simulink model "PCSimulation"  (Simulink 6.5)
settings: Solver=FixedStepDiscrete  SolverMode=SingleTasking  StartTime=0.0  StopTime=inf  FixedStep=samplePeriod  RelTol=1e-3  AbsTol=1e-6
PreLoadFcn:
  | initialize
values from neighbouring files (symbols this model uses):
  accelCanon = 9810    [initialize.m]
  accelFreq = inf    [initialize.m]
  actParams = [	bulkModulus   * pressCanon    [initialize.m]    (also in Copy of initialize.m)
  aFnd = [1]    [initialize.m]
  aFwd = [1]    [initialize.m]
  aLpf = [1]    [randth.m]
  bFnd = [1]    [initialize.m]
  bFwd = [1]    [initialize.m]
  bLpf = [1]    [randth.m]
  displFreq = inf    [initialize.m]
  flowCanon = 1.666667e+04    (= 16666.67)    [initialize.m]    (also in Copy of initialize.m)
  forceCanon = 1    [initialize.m]    (also in Copy of initialize.m)
  forceFreq = inf    [initialize.m]
  friction = 5			 				* 0.155000	 				* 0.00444822 				* area1    (= 2.71252900422)    [initialize.m]
  fsamp = 1 / samplePeriod    (= 1024)    [initialize.m]    (also in rampth.m = 1 / deltaT; randth.m = 1 / deltaT; rspect.m = 1.0 / tsamp; Copy of initialize.m)
  gasConstant = 1.8    [initialize.m]    (also in Copy of initialize.m)
  invFoundMass = 0.0    (= 0)    [initialize.m]
  invRigidMass = 0.0    (= 0)    [initialize.m]
  lengthCanon = 1    [initialize.m]    (also in Copy of initialize.m)
  maxDispl = ( (stroke2 + endLength2) * lengthCanon)'    [initialize.m]    (also in Copy of initialize.m)
  maxOilVolume = volume * (1 - (precharge/supplyPress)^(1/gasConstant))    (= 211.391477114)    [initialize.m]    (also in Copy of initialize.m)
  maxVeloc = ( (maxFlow' * flowCanon ./ (area1 * areaCanon)) / velocCanon)'    [initialize.m]    (also in rampth.m = 2 * maxDispl / (nVeloc * deltaT); Copy of initialize.m)
  minDispl = (-(stroke1 + endLength1) * lengthCanon)'    [initialize.m]    (also in Copy of initialize.m)
  minVeloc = (-(maxFlow' * flowCanon ./ (area2 * areaCanon)) / velocCanon)'    [initialize.m]    (also in Copy of initialize.m)
  nAdcU = 6    [initialize.m]    (also in Copy of initialize.m)
  nUDPInp = 1+6*nAct+nAdcU+nDucU+nEncU+nDout    (= 46)    [initialize.m]    (also in Copy of initialize.m)
  nUDPOut = 1+7*nAct+nAdcU+nDucU+nEncU+nDinp    (= 51)    [initialize.m]    (also in Copy of initialize.m)
  precharge = 3000		 				* 6.894757e-03    (= 20.684271)    [initialize.m]    (also in Copy of initialize.m)
  pumpFlow = 1e20    (= 1e+20)    [initialize.m]    (also in Copy of initialize.m)
  returnPress = 3			 				* 0.1    (= 0.3)    [initialize.m]    (also in Copy of initialize.m)
  samplePeriod = controlPeriod/upsampleFactor    (= 0.0009765625)    [initialize.m]    (also in viewer.m = eval(getHeaderValue(header, 'DELTA_T')); Copy of initialize.m)
  supplyPress = 280		 				* 0.1    (= 28)    [initialize.m]    (also in Copy of initialize.m)
  upsampleFactor = 1    [initialize.m]    (also in Copy of initialize.m)
  velocCanon = 1    [initialize.m]    (also in Copy of initialize.m)
  volume = 15.15		 				+ (  45		 				    * 2		 				   + 30		 				    * 6 )	 				* 5    (= 1365.15)    [initialize.m]    (also in quake.m = volume / 231.0; Copy of initialize.m)
  volumeCanon = 1e+06    (= 1000000)    [initialize.m]    (also in Copy of initialize.m)
  yieldDispl = 1.0    (= 1)    [initialize.m]
undefined symbols (not defined in the file or in its folder): DiscIntNeverNeededParam
libraries: simulink x1

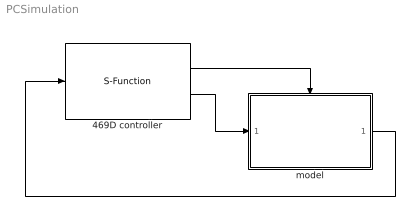
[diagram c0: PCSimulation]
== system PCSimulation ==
  469D controller : S-Function  FunctionName=ConnectUdpSimulink  Parameters=5002,nUDPInp,nUDPOut,upsampleFactor
  model : Subsystem  TreatAsAtomicUnit=on
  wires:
  model/1(out) -> 469D controller/1
  469D controller/1 -> model/Trigger
  469D controller/2 -> model/1(inp)

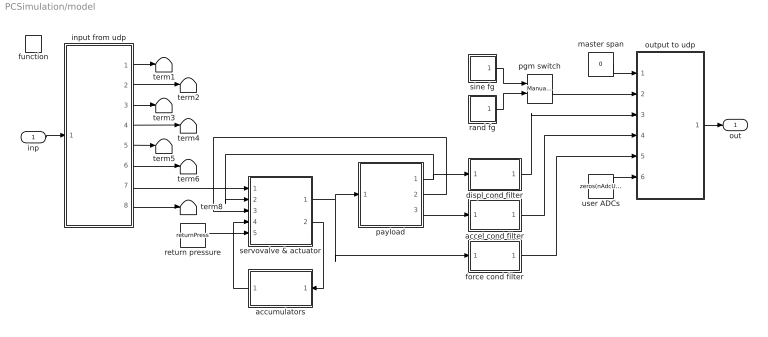
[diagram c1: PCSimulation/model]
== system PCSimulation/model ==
  inp : Inport
  function : TriggerPort  TriggerType=function-call
  accel cond filter : Subsystem  mask{freq3dB=accelFreq, fsamp=fsamp}
      mask prompts: freq3dB "3 dB cutoff frequency (inf, 500, 300, 100, 50 Hz)"; fsamp "Sampling frequency (Hz)"
      mask init:
      | if isempty(freq3dB)
      | 	freq3dB = fsamp;
      | elseif freq3dB == 500
      | 	freq3dB = 485;
      | elseif freq3dB == 300
      | 	freq3dB = 204.9;
      | elseif freq3dB == 100
      | 	freq3dB = 56.5;
      | elseif freq3dB == 50
      | 	freq3dB = 27.8;
      | else
      | 	freq3dB = fsamp;
      | end
      | if freq3dB > fsamp/2
      | 	a = [1];
      | 	b = [1];
      | else
      | 	[b, a] = ellip(4, 0.001, 60.0, 2*freq3dB/fsamp);
      | end
  accumulators : Subsystem  Orientation=left
  displ cond filter : Subsystem  mask{freq3dB=displFreq, fsamp=fsamp}
      mask prompts: freq3dB "3 dB cutoff frequency (inf, 500, 300, 100, 50 Hz)"; fsamp "Sampling frequency (Hz)"
      mask init:
      | if isempty(freq3dB)
      | 	freq3dB = fsamp;
      | elseif freq3dB == 500
      | 	freq3dB = 485;
      | elseif freq3dB == 300
      | 	freq3dB = 204.9;
      | elseif freq3dB == 100
      | 	freq3dB = 56.5;
      | elseif freq3dB == 50
      | 	freq3dB = 27.8;
      | else
      | 	freq3dB = fsamp;
      | end
      | if freq3dB > fsamp/2
      | 	a = [1];
      | 	b = [1];
      | else
      | 	[b, a] = ellip(4, 0.001, 60.0, 2*freq3dB/fsamp);
      | end
  force cond filter : Subsystem  mask{freq3dB=forceFreq, fsamp=fsamp}
      mask prompts: freq3dB "3 dB cutoff frequency (inf, 500, 300, 100, 50 Hz)"; fsamp "Sampling frequency (Hz)"
      mask init:
      | if isempty(freq3dB)
      | 	freq3dB = fsamp;
      | elseif freq3dB == 500
      | 	freq3dB = 485;
      | elseif freq3dB == 300
      | 	freq3dB = 204.9;
      | elseif freq3dB == 100
      | 	freq3dB = 56.5;
      | elseif freq3dB == 50
      | 	freq3dB = 27.8;
      | else
      | 	freq3dB = fsamp;
      | end
      | if freq3dB > fsamp/2
      | 	a = [1];
      | 	b = [1];
      | else
      | 	[b, a] = ellip(4, 0.001, 60.0, 2*freq3dB/fsamp);
      | end
  input from udp : Subsystem
  master span : Constant  Value=0  OutDataType=sfix(16)  ConRadixGroup=Use specified scaling  OutScaling=2^0  SampleTime=inf  FramePeriod=inf
  output to udp : Subsystem
  payload : Subsystem
  pgm switch : simulink/Signal Routing/Manual Switch  SystemSampleTime=-1  sw=0  action=0
  rand fg : Subsystem  mask(Sine Function Generator){ampl=1, bw=10, spanInterval=1, samplePeriod=samplePeriod}
      mask prompts: ampl "RMS amplitude"; bw "Bandwidth (Hz)"; spanInterval "Span interval (sec)"; samplePeriod "Sample period (sec)"
      mask init:
      | gain = ampl*sqrt(3)*sqrt(1/(2*samplePeriod*bw));
  return pressure : Constant  Value=returnPress  OutDataType=sfix(16)  ConRadixGroup=Use specified scaling  OutScaling=2^0  SampleTime=inf  FramePeriod=inf
  servovalve & actuator : Subsystem  mask(Actuator){params=actParams}
      mask prompts: params "Parameter vector"
  sine fg : Subsystem  mask(Sine Function Generator){ampl=1, freq=1, spanInterval=1, samplePeriod=samplePeriod}
      mask prompts: ampl "Amplitude"; freq "Frequency (Hz)"; spanInterval "Span interval (sec)"; samplePeriod "Sample period (sec)"
  term{1..6,8} (7 alike) : Terminator
  user ADCs : Constant  Value=zeros(nAdcU, 1)  OutDataType=sfix(16)  ConRadixGroup=Use specified scaling  OutScaling=2^0  SampleTime=inf  FramePeriod=inf
  out : Outport
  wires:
  servovalve & actuator/2(flow) -> accumulators/1(flow)
  accumulators/1(press) -> servovalve & actuator/4(spl press)
  return pressure/1 -> servovalve & actuator/5(rtn press)
  payload/1(displ) -> displ cond filter/1(inp), servovalve & actuator/2(displ)
  payload/2(veloc) -> servovalve & actuator/3(veloc)
  servovalve & actuator/1(force) -> payload/1(force), force cond filter/1(inp)
  payload/3(accel) -> accel cond filter/1(inp)
  inp/1 -> input from udp/1(inp)
  output to udp/1(out) -> out/1
  user ADCs/1 -> output to udp/6(user adcs)
  input from udp/1(master span) -> term1/1
  input from udp/2(ref) -> term2/1
  input from udp/3(displ fbk) -> term3/1
  input from udp/4(veloc fbk) -> term4/1
  input from udp/5(accel fbk) -> term5/1
  input from udp/6(force fbk) -> term6/1
  input from udp/7(valve cmd) -> servovalve & actuator/1(cmd)
  force cond filter/1(out) -> output to udp/5(force fbk)
  displ cond filter/1(out) -> output to udp/3(displ fbk)
  master span/1 -> output to udp/1(master span)
  sine fg/1(out) -> pgm switch/1
  rand fg/1(out) -> pgm switch/2
  pgm switch/1 -> output to udp/2(ref)
  input from udp/8(user adcs) -> term8/1
  accel cond filter/1(out) -> output to udp/4(accel fbk)

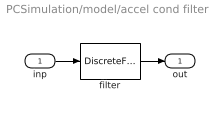
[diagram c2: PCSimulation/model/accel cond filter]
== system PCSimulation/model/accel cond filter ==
  inp : Inport
  filter : DiscreteFilter  Numerator=b  Denominator=a  SampleTime=-1
  out : Outport
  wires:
  inp/1 -> filter/1
  filter/1 -> out/1

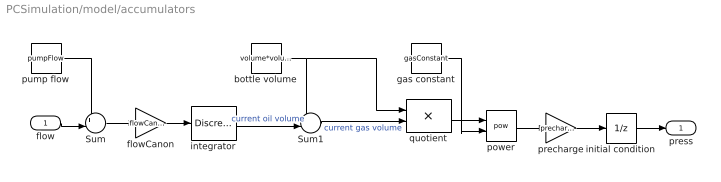
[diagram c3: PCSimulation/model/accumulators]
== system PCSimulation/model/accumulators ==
  flow : Inport
  Sum : Sum  Inputs=+-|
  Sum1 : Sum  Inputs=+-|
  bottle volume : Constant  Value=volume*volumeCanon  OutDataType=sfix(16)  ConRadixGroup=Use specified scaling  OutScaling=2^0  SampleTime=inf  FramePeriod=inf
  flowCanon : Gain  Gain=flowCanon
  gas constant : Constant  Value=gasConstant  OutDataType=sfix(16)  ConRadixGroup=Use specified scaling  OutScaling=2^0  SampleTime=inf  FramePeriod=inf
  initial condition : UnitDelay  X0=supplyPress  SampleTime=-1
  integrator : DiscreteIntegrator  InitialCondition=maxOilVolume*volumeCanon  SampleTime=-1  LimitOutput=on  UpperSaturationLimit=maxOilVolume*volumeCanon  LowerSaturationLimit=0  ICPrevOutput=DiscIntNeverNeededParam  ICPrevScaledInput=DiscIntNeverNeededParam
  power : Math  Operator=pow
  precharge : Gain  Gain=precharge
  pump flow : Constant  Value=pumpFlow  OutDataType=sfix(16)  ConRadixGroup=Use specified scaling  OutScaling=2^0  SampleTime=inf  FramePeriod=inf
  quotient : Product  Inputs=*/
  press : Outport
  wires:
  initial condition/1 -> press/1
  flowCanon/1 -> integrator/1
  flow/1 -> Sum/2
  integrator/1 -> Sum1/2  "current oil volume"
  quotient/1 -> power/1
  Sum1/1 -> quotient/2  "current gas volume"
  precharge/1 -> initial condition/1
  power/1 -> precharge/1
  gas constant/1 -> power/2
  bottle volume/1 -> quotient/1, Sum1/1
  Sum/1 -> flowCanon/1
  pump flow/1 -> Sum/1

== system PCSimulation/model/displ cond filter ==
  inp : Inport
  filter : DiscreteFilter  Numerator=b  Denominator=a  SampleTime=-1
  out : Outport
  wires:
  inp/1 -> filter/1
  filter/1 -> out/1

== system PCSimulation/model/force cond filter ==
  inp : Inport
  filter : DiscreteFilter  Numerator=b  Denominator=a  SampleTime=-1
  out : Outport
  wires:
  filter/1 -> out/1
  inp/1 -> filter/1

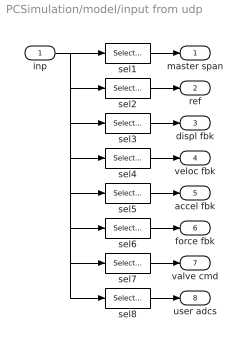
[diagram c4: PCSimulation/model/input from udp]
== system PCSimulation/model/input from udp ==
  inp : Inport
  sel1 : Selector  InputType=Vector  ElementSrc=Internal  Elements=1  RowSrc=Internal  Rows=1  ColumnSrc=Internal  Columns=1  InputPortWidth=nUDPOut  IndexIsStartValue=off
  sel2 : Selector  InputType=Vector  ElementSrc=Internal  Elements=2  RowSrc=Internal  Rows=1  ColumnSrc=Internal  Columns=1  InputPortWidth=nUDPOut  IndexIsStartValue=off
  sel3 : Selector  InputType=Vector  ElementSrc=Internal  Elements=3  RowSrc=Internal  Rows=1  ColumnSrc=Internal  Columns=1  InputPortWidth=nUDPOut  IndexIsStartValue=off
  sel4 : Selector  InputType=Vector  ElementSrc=Internal  Elements=4  RowSrc=Internal  Rows=1  ColumnSrc=Internal  Columns=1  InputPortWidth=nUDPOut  IndexIsStartValue=off
  sel5 : Selector  InputType=Vector  ElementSrc=Internal  Elements=5  RowSrc=Internal  Rows=1  ColumnSrc=Internal  Columns=1  InputPortWidth=nUDPOut  IndexIsStartValue=off
  sel6 : Selector  InputType=Vector  ElementSrc=Internal  Elements=6  RowSrc=Internal  Rows=1  ColumnSrc=Internal  Columns=1  InputPortWidth=nUDPOut  IndexIsStartValue=off
  sel7 : Selector  InputType=Vector  ElementSrc=Internal  Elements=7  RowSrc=Internal  Rows=1  ColumnSrc=Internal  Columns=1  InputPortWidth=nUDPOut  IndexIsStartValue=off
  sel8 : Selector  InputType=Vector  ElementSrc=Internal  Elements=8:12  RowSrc=Internal  Rows=1  ColumnSrc=Internal  Columns=1  InputPortWidth=nUDPOut  IndexIsStartValue=off
  master span : Outport
  ref : Outport  Port=2
  displ fbk : Outport  Port=3
  veloc fbk : Outport  Port=4
  accel fbk : Outport  Port=5
  force fbk : Outport  Port=6
  valve cmd : Outport  Port=7
  user adcs : Outport  Port=8
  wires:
  inp/1 -> sel1/1, sel2/1, sel3/1, sel4/1, sel5/1, sel6/1, sel7/1, sel8/1
  sel7/1 -> valve cmd/1
  sel6/1 -> force fbk/1
  sel5/1 -> accel fbk/1
  sel4/1 -> veloc fbk/1
  sel3/1 -> displ fbk/1
  sel2/1 -> ref/1
  sel1/1 -> master span/1
  sel8/1 -> user adcs/1

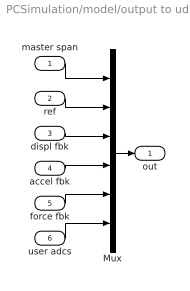
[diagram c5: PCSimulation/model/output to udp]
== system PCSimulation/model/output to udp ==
  master span : Inport
  ref : Inport  Port=2
  displ fbk : Inport  Port=3
  accel fbk : Inport  Port=4
  force fbk : Inport  Port=5
  user adcs : Inport  Port=6
  Mux : Mux  Inputs=6
  out : Outport
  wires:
  Mux/1 -> out/1
  master span/1 -> Mux/1
  ref/1 -> Mux/2
  displ fbk/1 -> Mux/3
  accel fbk/1 -> Mux/4
  force fbk/1 -> Mux/5
  user adcs/1 -> Mux/6

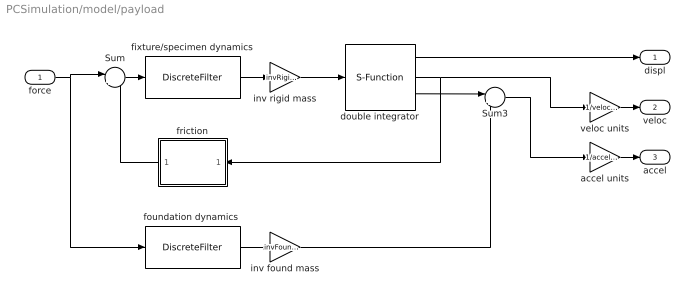
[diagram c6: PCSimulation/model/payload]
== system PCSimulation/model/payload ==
  force : Inport
  Sum : Sum  Inputs=|+-
  Sum3 : Sum  Inputs=|+-
  accel units : Gain  Gain=1/accelCanon
  double integrator : S-Function  FunctionName=doubleintegrator  Parameters=maxDispl, minDispl, initDispl, maxVeloc, minVeloc, initVeloc, samplePeriod  mask(Double integrator){maxDispl=maxDispl, minDispl=minDispl, initDispl=0, maxVeloc=maxVeloc*velocCanon, minVeloc=minVeloc*velocCanon, initVeloc=0, samplePeriod=samplePeriod}
      mask prompts: maxDispl "Maximum displacement"; minDispl "Minimum displacement"; initDispl "Initial displacement"; maxVeloc "Maximum velocity"; minVeloc "Minimum velocity"; initVeloc "Initial velocity"; samplePeriod "Sample period (sec)"
      mask help: Integrates acceleration twice to produce velocity and displacement. When clipping occurs, acceleration, velocity and displacement are adjusted accordingly.
  fixture/specimen dynamics : DiscreteFilter  Numerator=bFwd  Denominator=aFwd  SampleTime=-1
  "foundation dynamics " : DiscreteFilter  Numerator=bFnd  Denominator=aFnd  SampleTime=-1
  friction : Subsystem  Orientation=left  mask{friction=friction*forceCanon, yieldDispl=yieldDispl*lengthCanon, hysteresis=0}
      mask prompts: friction "Sliding friction"; yieldDispl "Equiv. yield displacement (in)"; hysteresis "Hysteresis constant"
  inv found mass : Gain  Gain=invFoundMass
  inv rigid mass : Gain  Gain=invRigidMass
  veloc units : Gain  Gain=1/velocCanon
  displ : Outport
  veloc : Outport  Port=2
  accel : Outport  Port=3
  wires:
  Sum/1 -> fixture/specimen dynamics/1
  veloc units/1 -> veloc/1
  friction/1(force) -> Sum/2
  force/1 -> Sum/1, "foundation dynamics "/1
  accel units/1 -> accel/1
  "foundation dynamics "/1 -> inv found mass/1
  inv found mass/1 -> Sum3/2
  fixture/specimen dynamics/1 -> inv rigid mass/1
  inv rigid mass/1 -> double integrator/1
  double integrator/3 -> Sum3/1
  double integrator/1 -> displ/1
  Sum3/1 -> accel units/1
  double integrator/2 -> friction/1(veloc), veloc units/1

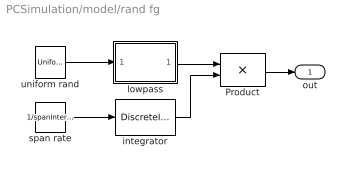
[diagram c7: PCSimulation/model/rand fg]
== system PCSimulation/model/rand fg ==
  Product : Product
  integrator : DiscreteIntegrator  SampleTime=-1  LimitOutput=on  UpperSaturationLimit=1  LowerSaturationLimit=0  ICPrevOutput=DiscIntNeverNeededParam  ICPrevScaledInput=DiscIntNeverNeededParam
  lowpass : Subsystem  mask{freq=bw, k=gain, samplePeriod=samplePeriod}
      mask prompts: freq "Cutoff frequency (Hz)"; k "Gain"; samplePeriod "Sample period (sec)"
      mask init:
      | damp = sqrt(2);
      | b = [0 0 (2*pi*freq)^2];
      | a = [1 2*(2*pi*freq)*damp (2*pi*freq)^2];
      | [bLpf aLpf] = bilinear(b, a, 1/samplePeriod);
  span rate : Constant  Value=1/spanInterval  OutDataType=sfix(16)  ConRadixGroup=Use specified scaling  OutScaling=2^0  SampleTime=inf  FramePeriod=inf
  uniform rand : UniformRandomNumber
  out : Outport
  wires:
  lowpass/1(out) -> Product/1
  uniform rand/1 -> lowpass/1(inp)
  Product/1 -> out/1
  span rate/1 -> integrator/1
  integrator/1 -> Product/2

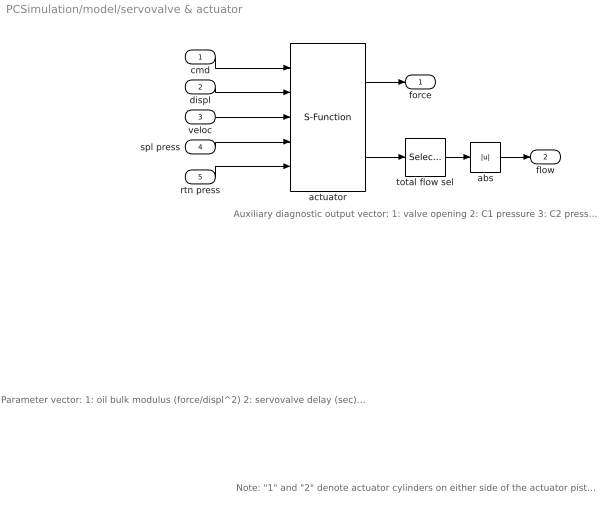
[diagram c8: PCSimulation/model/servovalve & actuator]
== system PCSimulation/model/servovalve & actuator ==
  note: Parameter vector: 1: oil bulk modulus (force/displ^2) 2: servovalve delay (sec) 3: servovalve overlap 4: rated pressure (force/displ^2) 5: rated flow at rated pressure (displ^3/sec) 6: nominal flow at rated pressure (displ^3/sec) 7: actuator piston area 1 (displ^2) 8: actuator piston area 2 (displ^2) 9: actuator usable stroke 1 (displ) 10: actuator usable stroke 2 (displ) 11: actuator end cushion length 1 (displ) 12: actuator end cushion length 2 (displ) 13: additional port volume 1 (displ^3) 14: additional port volume 1 (displ^3) 15: actuator parasitic damping factor 16: cross-chamber leakage factor (flow/press) 17: ratio port openings according to area 18: sample period (sec) Conversion factors used for converting signals from external (user) to internal (canonical) units: 19: displacement 20: velocity 21: force 22: pressure 23: flow
  note: Note: "1" and "2" denote actuator cylinders on either side of the actuator piston. With positive valve drive, oil is ported into cylinder 1, resulting in positive displacement.
  note: Auxiliary diagnostic output vector: 1: valve opening 2: C1 pressure 3: C2 pressure 4: delta pressure 5: force 6: velocity 7: C1 flow 8: C2 flow 9: total flow 10: kinematic flow 11: compressibility flow 12: leakage flow 13: C1 oilspring displacement 14: C2 oilspring displacement 15: C1 oilspring velocity 16: C2 oilspring velocity
  cmd : Inport
  displ : Inport  Port=2
  veloc : Inport  Port=3
  spl press : Inport  Port=4
  rtn press : Inport  Port=5
  abs : Abs  SaturateOnIntegerOverflow=on  SampleTime=-1
  actuator : S-Function  FunctionName=Actuator  Parameters=params
  total flow sel : Selector  InputType=Vector  ElementSrc=Internal  Elements=9  RowSrc=Internal  Rows=1  ColumnSrc=Internal  Columns=1  IndexIsStartValue=off
  force : Outport
  flow : Outport  Port=2
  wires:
  spl press/1 -> actuator/4
  rtn press/1 -> actuator/5
  cmd/1 -> actuator/1
  actuator/1 -> force/1
  displ/1 -> actuator/2
  veloc/1 -> actuator/3
  actuator/2 -> total flow sel/1
  total flow sel/1 -> abs/1
  abs/1 -> flow/1

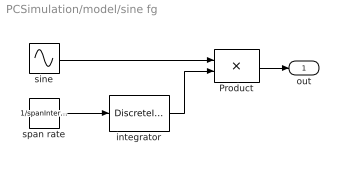
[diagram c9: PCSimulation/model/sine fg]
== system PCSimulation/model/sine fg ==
  Product : Product
  integrator : DiscreteIntegrator  SampleTime=-1  LimitOutput=on  UpperSaturationLimit=1  LowerSaturationLimit=0  ICPrevOutput=DiscIntNeverNeededParam  ICPrevScaledInput=DiscIntNeverNeededParam
  sine : Sin  Amplitude=ampl  Frequency=2 * pi * freq
  span rate : Constant  Value=1/spanInterval  OutDataType=sfix(16)  ConRadixGroup=Use specified scaling  OutScaling=2^0  SampleTime=inf  FramePeriod=inf
  out : Outport
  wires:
  integrator/1 -> Product/2
  span rate/1 -> integrator/1
  sine/1 -> Product/1
  Product/1 -> out/1

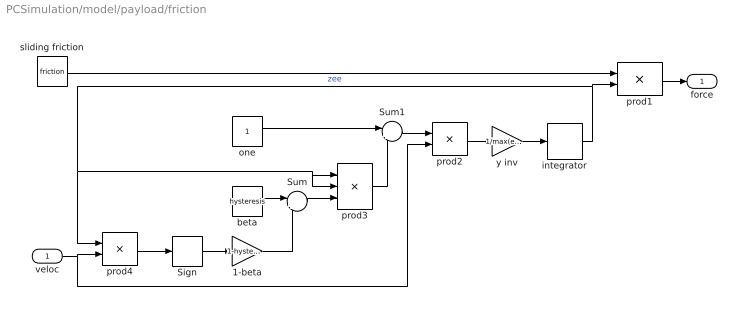
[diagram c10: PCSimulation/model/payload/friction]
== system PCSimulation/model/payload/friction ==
  veloc : Inport
  1-beta : Gain  Gain=1-hysteresis
  Sign : Signum
  Sum : Sum  Inputs=|++
  Sum1 : Sum  Inputs=|+-
  beta : Constant  Value=hysteresis  OutDataType=sfix(16)  ConRadixGroup=Use specified scaling  OutScaling=2^0  SampleTime=inf  FramePeriod=inf
  integrator : DiscreteIntegrator  SampleTime=-1  LimitOutput=on  UpperSaturationLimit=1  LowerSaturationLimit=-1  ICPrevOutput=DiscIntNeverNeededParam  ICPrevScaledInput=DiscIntNeverNeededParam
  one : Constant  Value=1  OutDataType=sfix(16)  ConRadixGroup=Use specified scaling  OutScaling=2^0  SampleTime=inf  FramePeriod=inf
  prod1 : Product
  prod2 : Product
  prod3 : Product  Inputs=3
  prod4 : Product
  sliding friction : Constant  Value=friction  OutDataType=sfix(16)  ConRadixGroup=Use specified scaling  OutScaling=2^0  SampleTime=inf  FramePeriod=inf
  y inv : Gain  Gain=1/max(eps, yieldDispl)
  force : Outport
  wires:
  integrator/1 -> prod3/2, prod3/1, prod4/1, prod1/2  "zee"
  y inv/1 -> integrator/1
  prod2/1 -> y inv/1
  Sum1/1 -> prod2/1
  prod3/1 -> Sum1/2
  one/1 -> Sum1/1
  Sum/1 -> prod3/3
  beta/1 -> Sum/1
  1-beta/1 -> Sum/2
  Sign/1 -> 1-beta/1
  prod4/1 -> Sign/1
  veloc/1 -> prod2/2, prod4/2
  prod1/1 -> force/1
  sliding friction/1 -> prod1/1

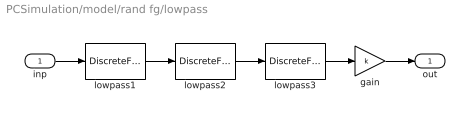
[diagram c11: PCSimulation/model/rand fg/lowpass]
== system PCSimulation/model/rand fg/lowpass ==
  inp : Inport
  gain : Gain  Gain=k
  lowpass1 : DiscreteFilter  Numerator=bLpf  Denominator=aLpf  SampleTime=-1
  lowpass2 : DiscreteFilter  Numerator=bLpf  Denominator=aLpf  SampleTime=-1
  lowpass3 : DiscreteFilter  Numerator=bLpf  Denominator=aLpf  SampleTime=-1
  out : Outport
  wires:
  lowpass3/1 -> gain/1
  lowpass2/1 -> lowpass3/1
  lowpass1/1 -> lowpass2/1
  gain/1 -> out/1
  inp/1 -> lowpass1/1
